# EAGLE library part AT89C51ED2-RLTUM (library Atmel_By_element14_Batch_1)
8-bit Flash Microcontroller
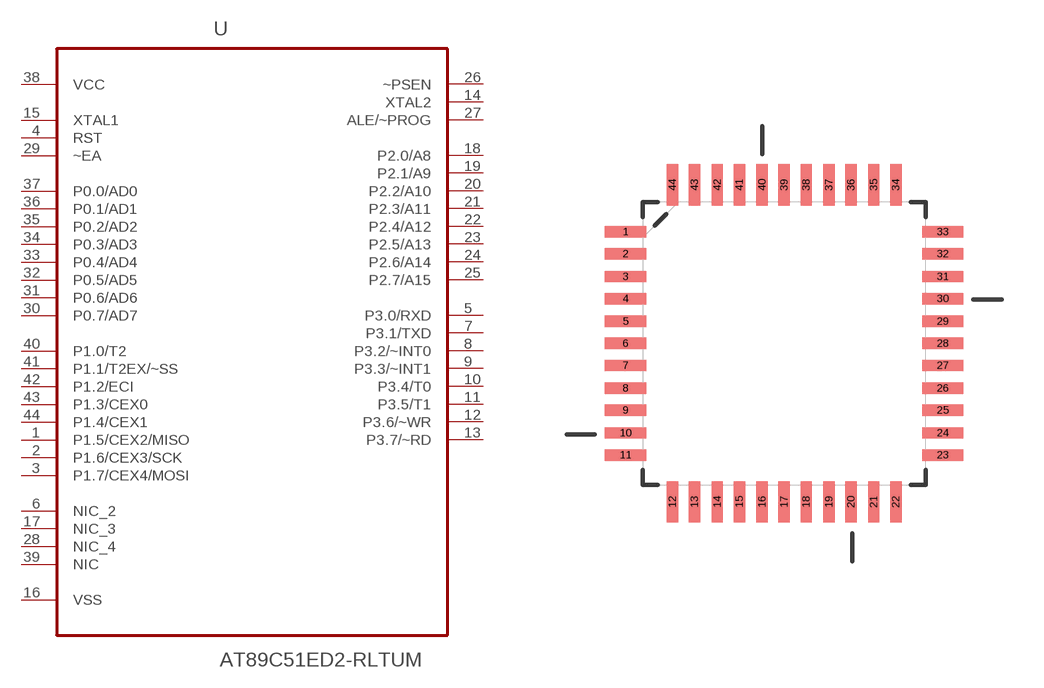
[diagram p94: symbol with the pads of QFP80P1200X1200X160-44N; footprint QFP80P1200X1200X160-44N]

Designator prefix U

## AT89C51ED2-RLTUM (DESCRIPTION: 8-bit Flash Microcontroller; MPN: AT89C51ED2-RLTUM; OC_FARNELL: 1095725; OC_NEWARK: 96K6567; PACKAGE: VQFP-44; SUPPLIER: ATMEL)  [QFP80P1200X1200X160-44N]
1  P1.5/CEX2/MISO
2  P1.6/CEX3/SCK
3  P1.7/CEX4/MOSI
4  RST  in
5  P3.0/RXD
6  NIC_2  nc
7  P3.1/TXD
8  P3.2/~INT0
9  P3.3/~INT1
10  P3.4/T0
11  P3.5/T1
12  P3.6/~WR
13  P3.7/~RD
14  XTAL2  out
15  XTAL1  in
16  VSS  pwr
17  NIC_3  nc
18  P2.0/A8
19  P2.1/A9
20  P2.2/A10
21  P2.3/A11
22  P2.4/A12
23  P2.5/A13
24  P2.6/A14
25  P2.7/A15
26  ~PSEN  out
27  ALE/~PROG  out
28  NIC_4  nc
29  ~EA  in
30  P0.7/AD7
31  P0.6/AD6
32  P0.5/AD5
33  P0.4/AD4
34  P0.3/AD3
35  P0.2/AD2
36  P0.1/AD1
37  P0.0/AD0
38  VCC  pwr
39  NIC  nc
40  P1.0/T2
41  P1.1/T2EX/~SS
42  P1.2/ECI
43  P1.3/CEX0
44  P1.4/CEX1

## Footprint QFP80P1200X1200X160-44N (pad centres in mm)
smd 1.473 x 0.406: 1 -5.664,3.988; 2 -5.664,3.2; 3 -5.664,2.388; 4 -5.664,1.6; 5 -5.664,0.787; 6 -5.664,0; 7 -5.664,-0.787; 8 -5.664,-1.6; 9 -5.664,-2.388; 10 -5.664,-3.2; 11 -5.664,-3.988; 23 5.664,-3.988; 24 5.664,-3.2; 25 5.664,-2.388; 26 5.664,-1.6; 27 5.664,-0.787; 28 5.664,0; 29 5.664,0.787; 30 5.664,1.6; 31 5.664,2.388; 32 5.664,3.2; 33 5.664,3.988
smd 0.406 x 1.473: 12 -3.988,-5.664; 13 -3.2,-5.664; 14 -2.388,-5.664; 15 -1.6,-5.664; 16 -0.787,-5.664; 17 0,-5.664; 18 0.787,-5.664; 19 1.6,-5.664; 20 2.388,-5.664; 21 3.2,-5.664; 22 3.988,-5.664; 34 3.988,5.664; 35 3.2,5.664; 36 2.388,5.664; 37 1.6,5.664; 38 0.787,5.664; 39 0,5.664; 40 -0.787,5.664; 41 -1.6,5.664; 42 -2.388,5.664; 43 -3.2,5.664; 44 -3.988,5.664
